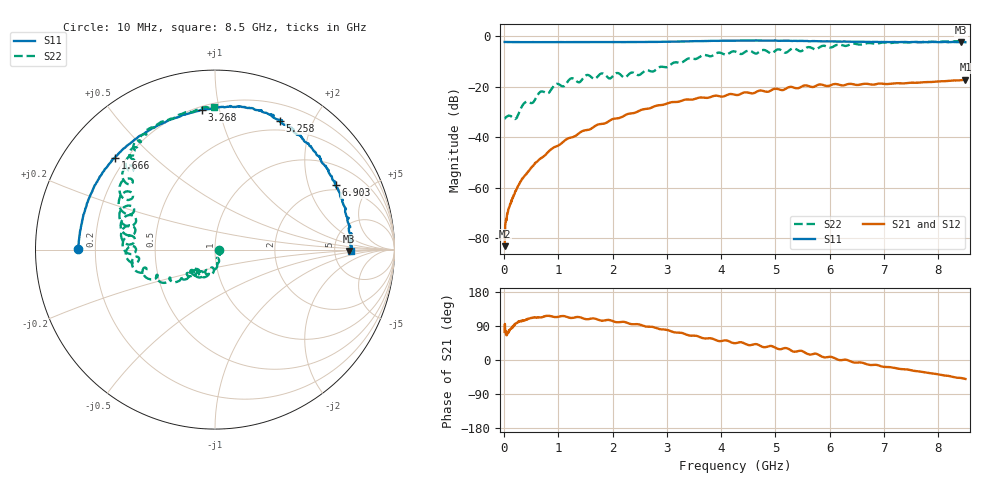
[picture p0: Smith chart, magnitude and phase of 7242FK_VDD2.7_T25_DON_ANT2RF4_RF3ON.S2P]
!Agilent Technologies,E5071C,MY46417908,A.11.23
!Date: Wed Dec 09 15:39:45 2020
!Data & Calibration Information:
!Freq	S11:SOLT2(ON)	S21:SOLT2(ON)	S12:SOLT2(ON)	S22:SOLT2(ON)
!PortZ  Port1:50+j0  Port2:50+j0
!Above PortZ is port z conversion or system Z0 setting when saving the data.
!When reading, reference impedance value at option line is always used.
# Hz S dB R 50
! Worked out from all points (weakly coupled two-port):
!   1601 points, 10 MHz to 8.5 GHz, reference 50 ohm
!   highest |S21| = -17.28 dB at 8.5 GHz (marker M1); lowest = -83.2 dB at 10 MHz (marker M2)
!   lowest |S11| = -2.5 dB at 8.415 GHz (marker M3), VSWR 6.94, Z = 347 - j11.2 ohm
!   |S11| at or under -10 dB: nowhere
!   |S22| runs from -32.9 to -2.0 dB; largest |S21 - S12| = 0.0021
!   S11 on the Smith chart (normalised r, x): 10 MHz: 0.13, +0.00; 1.666 GHz: 0.16, +0.38; 3.268 GHz: 0.22, +0.88; 5.258 GHz: 0.38, +1.55; 6.903 GHz: 1.76, +3.03; 8.5 GHz: 7.18, -0.18
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1e7  -2.34 179.7  -83.24 74.1  -84.50 71.1  -32.68 -1.5
1.108188e8  -2.38 176.8  -66.67 80.2  -66.38 78.7  -31.63 -38.6
2.2225e8  -2.40 173.7  -61.00 96.5  -60.96 96.4  -32.62 -46.4
3.655188e8  -2.42 169.6  -55.70 103.8  -55.63 105.0  -26.71 -58.7
5.247062e8  -2.40 165.4  -51.63 111.2  -51.63 111.5  -26.45 -73.4
6.626688e8  -2.43 161.9  -48.67 112.4  -48.69 112.7  -22.16 -77.7
8.112438e8  -2.40 158.2  -45.91 116.6  -45.92 116.6  -22.65 -86.5
9.598188e8  -2.41 154.3  -43.70 113.2  -43.72 113.1  -19.01 -92.9
1.426769e9  -2.40 143.5  -37.83 111.5  -37.83 111.4  -17.54 -104.6
1.532894e9  -2.40 140.6  -37.19 107.6  -37.20 107.6  -15.41 -116.3
1.66555e9  -2.41 137.4  -35.82 109.6  -35.83 109.5  -17.00 -120.1
2.482712e9  -2.37 115.4  -29.67 94.0  -29.67 94.0  -15.46 -135.5
2.843538e9  -2.32 105.5  -27.43 82.5  -27.43 82.6  -12.54 -135.0
3.268038e9  -2.12 95.4  -25.66 71.6  -25.67 71.6  -10.54 -146.8
4.255e9  -1.84 77.2  -23.26 44.4  -23.27 44.3  -6.12 -179.3
5.257881e9  -1.91 63.4  -20.20 28.0  -20.17 28.1  -5.63 164.8
5.671769e9  -2.01 53.4  -20.19 14.9  -20.13 14.7  -4.73 146.0
6.902819e9  -2.35 28.3  -18.82 -14.3  -18.85 -14.3  -2.87 128.9
7.088538e9  -2.36 23.8  -18.94 -18.5  -19.01 -18.4  -2.72 124.4
7.773044e9  -2.36 9.7  -18.26 -33.0  -18.27 -32.9  -2.28 114.2
8.4151e9  -2.52 -0.5  -17.49 -47.4  -17.58 -47.7  -2.00 93.2
8.5e9  -2.43 -0.4  -17.28 -50.0  -17.40 -49.9  -1.99 90.5
